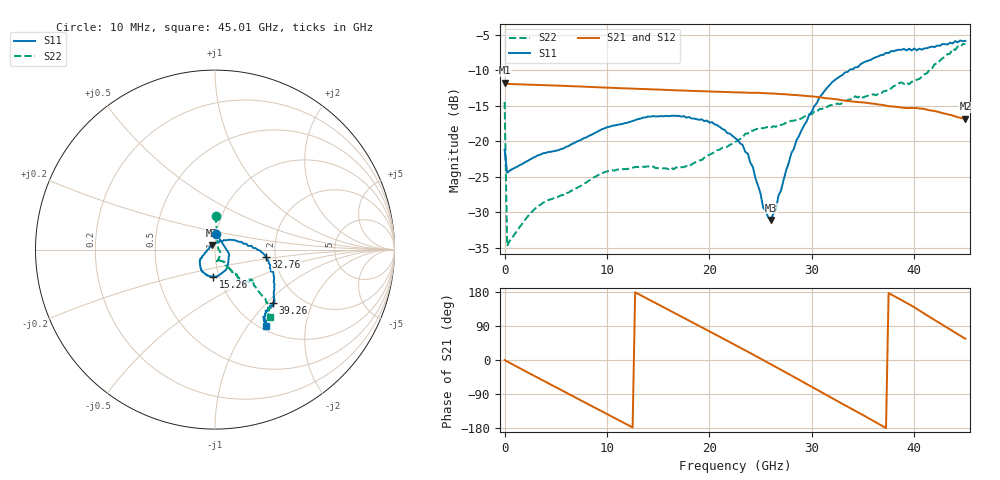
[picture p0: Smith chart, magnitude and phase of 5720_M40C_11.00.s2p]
! Device:  ADRF5720
! Description: 0.5dB LSB GaAs MMIC 6-bit Digital Attenuator
! Frequency:  0.000009 -  40 GHz
! Ports:
!	RF1	= Port 1
!	RF2	= Port 2
! Vdd:  3.3 Volt
! Vss:  -3.3 Volt
! Control:  0/3.3 Volt
! State:  11.00 dB attenuation
! Data:  The device was measured using G-S-G Probes on a matrix board.
!  Data was collected using an calibrated 4 port network analyzer.
!  The reference plane for this measurement is at the launchers.
! Note:  Analog Devices supplies this data as a sample of measured data
!  for this product.  Your particular data for this product may vary.
!  Data was taken at -40 degrees C.
!  Analog Devices reserves the right to change this data at anytime.
# GHZ S DB R 45.0
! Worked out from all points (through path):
!   181 points, 10 MHz to 45.01 GHz, reference 45 ohm
!   highest |S21| = -11.74 dB at 10 MHz (marker M1); lowest = -16.8 dB at 45.01 GHz (marker M2)
!   group delay of S21, straight-line fit = 40.6 ps
!   lowest |S11| = -31.1 dB at 26.01 GHz (marker M3), VSWR 1.06, Z = 43.5 + j1.99 ohm
!   |S11| at or under -10 dB: start of sweep to 33.66 GHz
!   |S22| runs from -34.8 to -6.3 dB; largest |S21 - S12| = 0.001
!   S11 on the Smith chart (normalised r, x): 10 MHz: 1.00, +0.17; 15.26 GHz: 0.94, -0.29; 32.76 GHz: 1.78, -0.16; 39.26 GHz: 1.47, -1.08; 45.01 GHz: 1.07, -1.22
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0.01  -21.20 85.0  -11.74 -0.1  -11.76 -0.1  -14.46 88.8
0.26  -24.44 7.1  -11.91 -3.9  -11.93 -4.0  -34.77 24.2
3.26  -21.97 -15.5  -12.06 -47.0  -12.09 -47.0  -29.11 -30.1
5.51  -21.09 -29.8  -12.17 -79.0  -12.19 -79.0  -27.61 -47.1
7.76  -19.55 -45.8  -12.30 -110.8  -12.32 -110.8  -25.97 -63.3
11.51  -17.54 -68.8  -12.52 -163.8  -12.54 -163.8  -23.92 -76.3
15.26  -16.44 -93.5  -12.72 143.2  -12.74 143.1  -23.82 -77.8
19.01  -16.97 -117.7  -12.92 89.9  -12.94 89.9  -22.69 -60.3
22.76  -19.80 -145.8  -13.10 36.3  -13.13 36.2  -19.92 -54.9
23.76  -21.73 -151.8  -13.15 21.8  -13.18 21.7  -18.89 -55.4
25.26  -29.33 173.2  -13.20 -0.1  -13.22 -0.2  -18.16 -54.0
26.01  -31.06 125.2  -13.26 -11.2  -13.29 -11.3  -18.09 -53.4
26.51  -29.65 87.5  -13.30 -18.7  -13.33 -18.8  -17.96 -54.1
26.76  -27.61 78.6  -13.34 -22.3  -13.36 -22.5  -17.66 -52.3
28.01  -21.68 38.9  -13.44 -40.9  -13.47 -41.0  -17.11 -53.3
30.26  -15.02 10.5  -13.70 -74.7  -13.73 -74.8  -15.82 -51.8
32.76  -10.86 -8.2  -14.16 -112.1  -14.18 -112.2  -14.78 -50.3
35.51  -8.64 -27.5  -14.61 -153.0  -14.63 -153.1  -13.57 -49.6
37.76  -7.29 -39.9  -15.09 173.0  -15.11 172.8  -12.56 -49.4
39.26  -7.19 -42.8  -15.32 150.9  -15.34 150.7  -11.69 -41.9
42.01  -6.73 -54.4  -15.74 105.3  -15.77 105.2  -9.13 -44.0
45.01  -5.85 -56.1  -16.82 56.0  -16.85 55.9  -6.27 -50.7
